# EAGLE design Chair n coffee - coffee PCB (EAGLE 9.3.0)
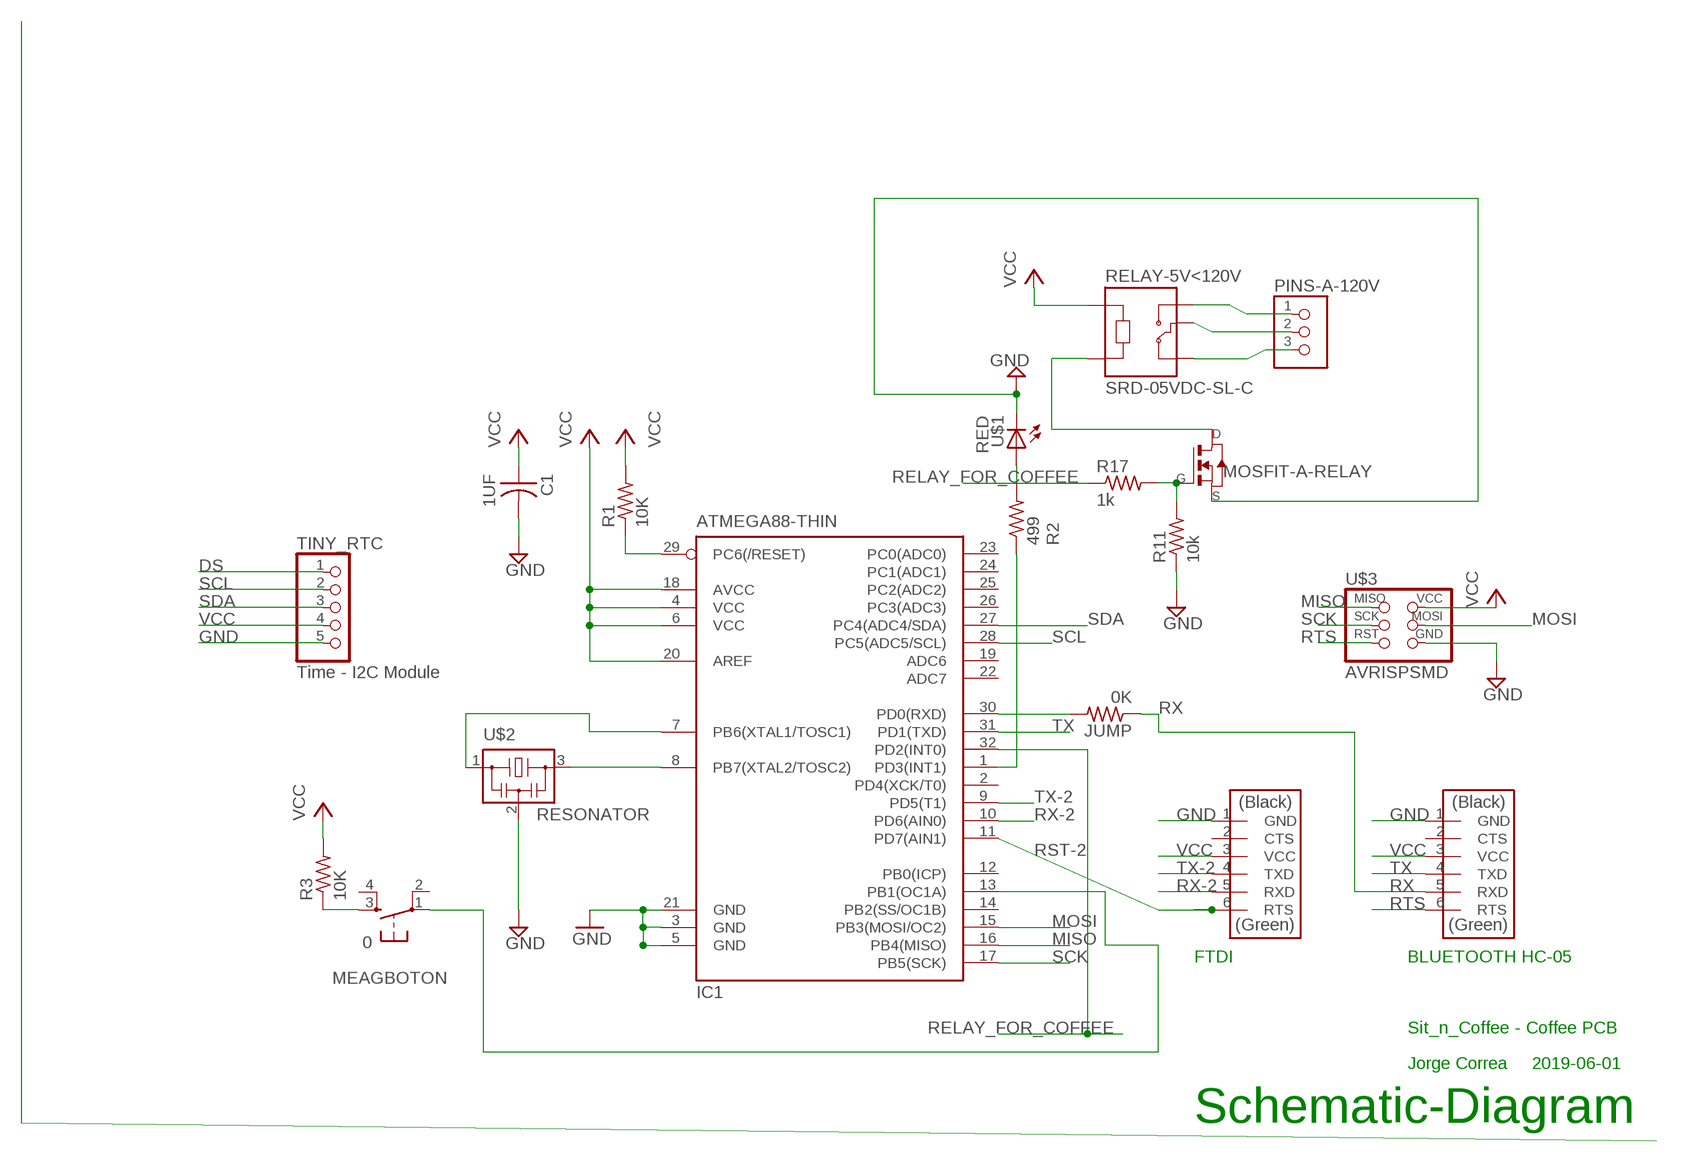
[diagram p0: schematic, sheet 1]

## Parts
C1  1UF  CAP-US1206FAB  [C1206FAB]
IC1  ATMEGA88-THIN  [TQFP32-08THIN]
JUMP  0K  RES-US1206FAB  [R1206FAB]
MEAGBOTON  0  6MM_SWITCH6MM_SWITCH  [6MM_SWITCH]
MOSFIT-A-RELAY  NMOSFETTO252  [TO252]
PINS-A-120V  TERM-1X03'-FABLAB'  [ED555DS-3DS]
R1  10K  RES-US1206FAB  [R1206FAB]
R2  499  RES-US1206FAB  [R1206FAB]
R3  10K  RES-US1206FAB  [R1206FAB]
R11  10k  RES-US1206FAB  [R1206FAB]
R17  1k  RES-US1206FAB  [R1206FAB]
RELAY-5V<120V  SRD-05VDC-SL-C  [RELAY_SRD-05VDC-SL-C]
TINY_RTC  Time - I2C Module  PINHD-1X5  [1X05]
U$1  RED  LEDFAB1206  [LED1206FAB]
U$2  RESONATOR  [EFOBM]
U$3  AVRISPSMD  [2X03SMD]
U$4  FTDI-SMD-HEADER  [1X06SMD]
U$5  FTDI-SMD-HEADER  [1X06SMD]

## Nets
DS: TINY_RTC.1
GND: C1.2 IC1.3(GND) IC1.5(GND) IC1.21(GND) MOSFIT-A-RELAY.2(S) R11.1 TINY_RTC.5 U$1.2(C) U$2.2 U$3.6(GND) U$4.1(GND) U$5.1(GND)
MISO: IC1.16(PB4(MISO)) U$3.1(MISO)
MOSI: IC1.15(PB3(MOSI/OC2)) U$3.4(MOSI)
N$1: IC1.8(PB7(XTAL2/TOSC2)) U$2.3
N$2: IC1.7(PB6(XTAL1/TOSC1)) U$2.1
N$3: IC1.29(PC6(/RESET)) R1.1
N$4: R2.2 U$1.1(A)
N$5: MEAGBOTON.3(S) R3.1
N$7: MOSFIT-A-RELAY.1(G) R11.2 R17.2
N$8: PINS-A-120V.2 RELAY-5V<120V.COM
N$9: PINS-A-120V.1 RELAY-5V<120V.NO
N$10: IC1.1(PD3(INT1)) R2.1
N$11: IC1.13(PB1(OC1A)) MEAGBOTON.1(P)
N$35: MOSFIT-A-RELAY.3(D) RELAY-5V<120V.A2
N$37: PINS-A-120V.3 RELAY-5V<120V.NC
RELAY_FOR_COFFEE: IC1.32(PD2(INT0)) R17.1
RST-2: IC1.11(PD7(AIN1)) U$4.6(RTS)
RTS: U$3.5(RST) U$5.6(RTS)
RX: IC1.30(PD0(RXD)) JUMP.1 JUMP.2 U$5.5(RXD)
RX-2: IC1.10(PD6(AIN0)) U$4.5(RXD)
SCK: IC1.17(PB5(SCK)) U$3.3(SCK)
SCL: IC1.28(PC5(ADC5/SCL)) TINY_RTC.2
SDA: IC1.27(PC4(ADC4/SDA)) TINY_RTC.3
TX: IC1.31(PD1(TXD)) U$5.4(TXD)
TX-2: IC1.9(PD5(T1)) U$4.4(TXD)
VCC: C1.1 IC1.4(VCC) IC1.6(VCC) IC1.18(AVCC) IC1.20(AREF) R1.2 R3.2 RELAY-5V<120V.A1 TINY_RTC.4 U$3.2(VCC) U$4.3(VCC) U$5.3(VCC)
Unconnected: IC1.2(PD4(XCK/T0)) IC1.12(PB0(ICP)) IC1.14(PB2(SS/OC1B)) IC1.19(ADC6) IC1.22(ADC7) IC1.23(PC0(ADC0)) IC1.24(PC1(ADC1)) IC1.25(PC2(ADC2)) IC1.26(PC3(ADC3)) MEAGBOTON.2(P1) MEAGBOTON.4(S1) U$4.2(CTS) U$5.2(CTS)

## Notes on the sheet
- FTDI | BLUETOOTH HC-05
- Sit_n_Coffee - Coffee PCB
- Jorge Correa | 2019-06-01
- Schematic-Diagram

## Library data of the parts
C1 = fab:CAP-US
IC1 = fab:ATMEGA88-THIN
JUMP R1-R3 R11 R17 = fab:RES-US: Resistor (US Symbol)
MEAGBOTON = fab:6MM_SWITCH: OMRON SWITCH
MOSFIT-A-RELAY = fab:NMOSFET: MOS FET
PINS-A-120V = fab:TERM-1X03: 3.5mm terminal block, 3 positions ED555-3DS as found in the fablab inventory. Made by Zaerc.
RELAY-5V<120V = SRD-05VDC-SL-C:SRD-05VDC-SL-C: 5V Trigger Relay Module For Arduino And Raspberry Pi 5V Trigger Relay Module For Arduino And Raspberry Pi; AVAILABILITY: Unavailable; DESCRIPTION: 5V Trigger Relay Module For Arduino And Raspberry Pi 5V Trigger Relay Module For Arduino And Raspberry Pi; MF: Songle Relay; MP: SRD-05VDC-SL-C; PACKAGE: None; PRICE: None
TINY_RTC = pinhead:PINHD-1X5: PIN HEADER
U$1 = fab:LED: LED
U$2 = fab:RESONATOR
U$3 = fab:AVRISP
U$4 U$5 = fab:FTDI-SMD-HEADER

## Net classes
0 default: width 0.508 mm, clearance 0.508 mm

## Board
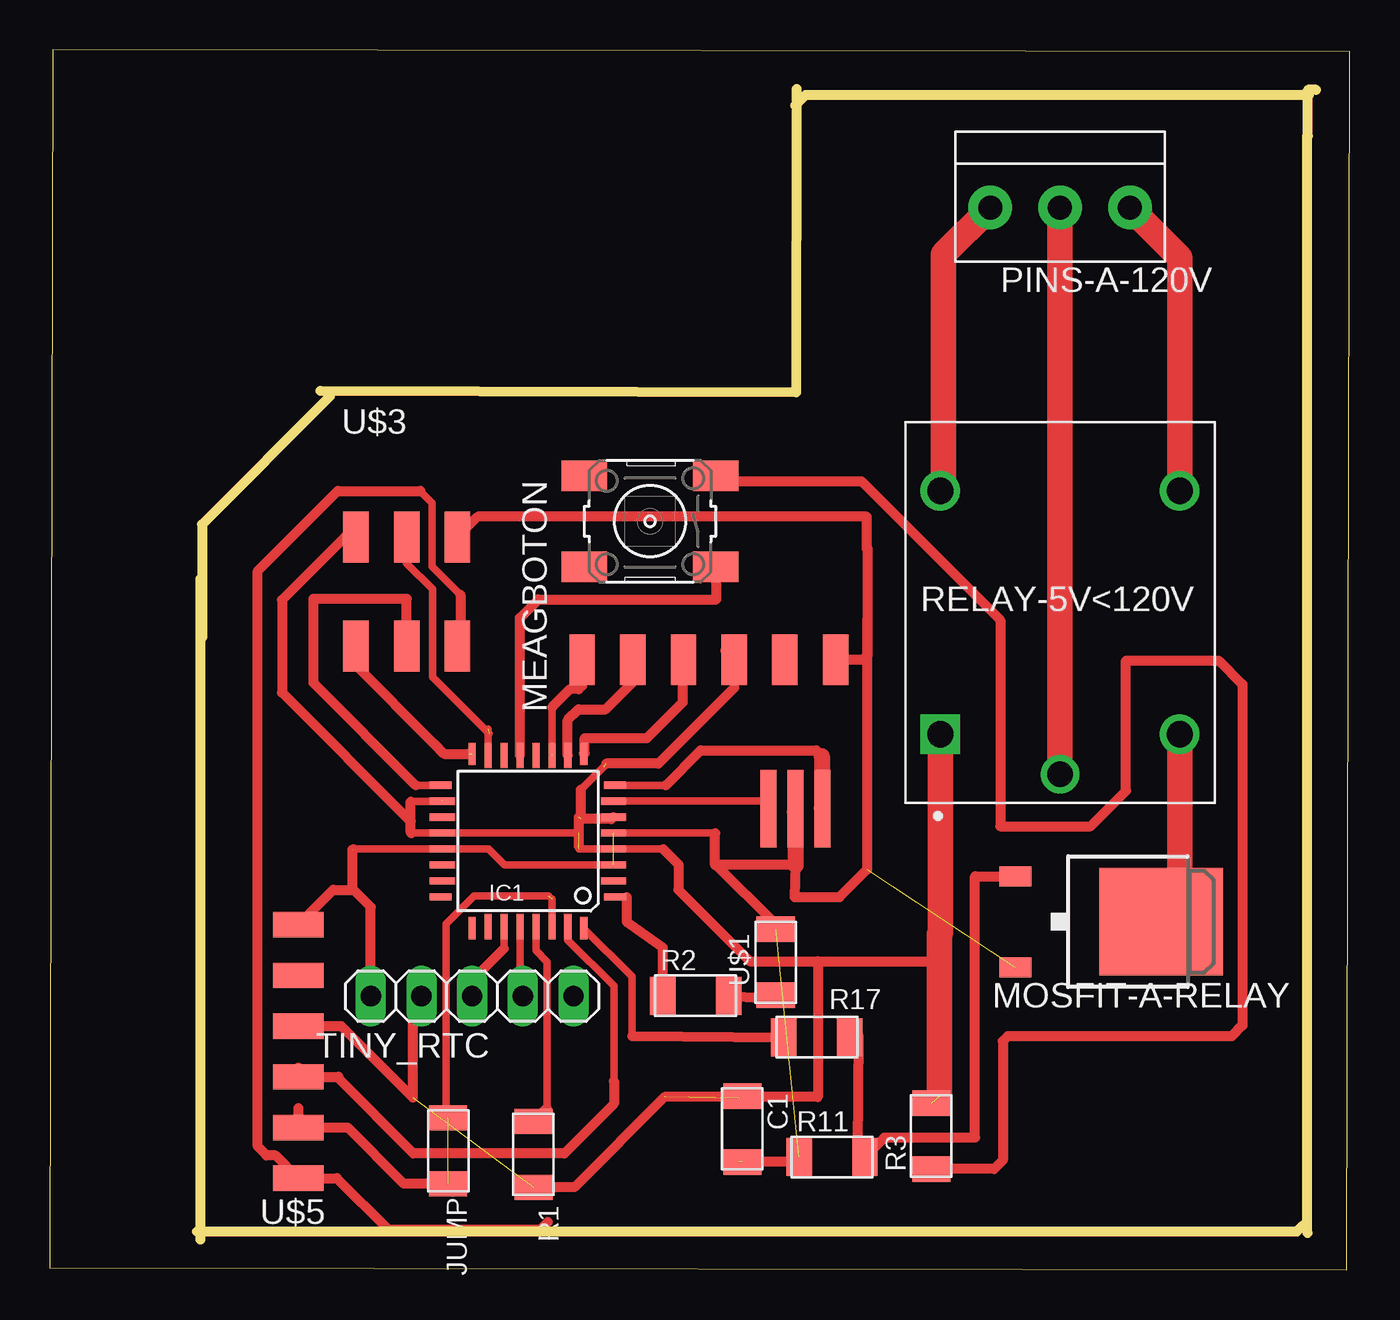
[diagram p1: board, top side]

Size 65.13 x 61.14 mm. Coordinates in mm from the lower left corner, seen from the top.
Outline: 0,0.1 64.98,0 65.13,61.04 0.15,61.14 0,0.1
Copper layers (1*16): Top 0.035mm / dielectric 1.5mm / Bottom 0.035mm
Design rules "default": minimum track width 6mil, minimum drill 0.35mm, track to track 6mil, track to pad 6mil, pad to pad 6mil, via to via 6mil, smd to smd 6mil, copper to edge 40mil, drill to drill 6mil, minimum pad ring 10mil, minimum via ring 8mil, stop-mask expansion 4mil, vias tented up to drill 0mil, thermal gap 10mil
Milling: 12 lines

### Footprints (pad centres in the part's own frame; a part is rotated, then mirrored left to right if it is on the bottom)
C1206FAB = smd 1.27 x 1.905: 1 -1.651,0; 2 1.651,0
TQFP32-08THIN = smd 1.118 x 0.356: 1 -4.369,2.8; 8 -4.369,-2.8; 17 4.369,-2.8; 24 4.369,2.8 | smd 1.27 x 0.356: 2 -4.293,2; 3 -4.293,1.2; 4 -4.293,0.4; 5 -4.293,-0.4; 6 -4.293,-1.2; 7 -4.293,-2; 18 4.293,-2; 19 4.293,-1.2; 20 4.293,-0.4; 21 4.293,0.4; 22 4.293,1.2; 23 4.293,2 | smd 0.356 x 1.118: 9 -2.8,-4.369; 16 2.8,-4.369; 25 2.8,4.369; 32 -2.8,4.369 | smd 0.356 x 1.27: 10 -2,-4.293; 14 1.2,-4.293; 15 2,-4.293; 26 2,4.293; 27 1.2,4.293; 31 -2,4.293 | smd 0.35 x 1.27: 11 -1.2,-4.293; 12 -0.4,-4.293; 13 0.4,-4.293; 28 0.4,4.293; 29 -0.4,4.293; 30 -1.2,4.293
R1206FAB = smd 1.27 x 1.905: 1 -1.651,0; 2 1.651,0
6MM_SWITCH = smd 2.286 x 1.524: 1 -3.302,2.286; 2 3.302,2.286; 3 -3.302,-2.286; 4 3.302,-2.286
TO252 = smd 1 x 1.6: 1 -2.28,-4.8; 2 2.28,-4.8 | smd 5.4 x 6.2: 3 0,2.5
ED555DS-3DS = drill 1.2 pad 2.184: 1 -3.5,0; 2 0,0; 3 3.5,0
RELAY_SRD-05VDC-SL-C = drill 1.32 square: A1 -6.1,6 | drill 1.32: A2 -6.1,-6; NC 6.1,6; NO 6.1,-6 | drill 1.29: COM -8.1,0
1X05 = drill 1.016 long: 1 -5.08,0; 2 -2.54,0; 3 0,0; 4 2.54,0; 5 5.08,0
LED1206FAB = smd 1.27 x 1.905: 1 -1.651,0; 2 1.651,0
EFOBM = smd 0.8 x 3.9: 1 -1.35,0; 2 0,0; 3 1.35,0
2X03SMD = smd 2.54 x 1.27: 1 -2.54,2.54; 2 2.92,2.54; 3 -2.54,0; 4 2.92,0; 5 -2.54,-2.54; 6 2.92,-2.54
1X06SMD = smd 2.54 x 1.27: 1 0,6.35; 2 0,3.81; 3 0,1.27; 4 0,-1.27; 5 0,-3.81; 6 0,-6.35

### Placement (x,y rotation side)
C1  34.7,7.06 270 top
IC1  23.95,21.49 180 top
JUMP  19.96,5.97 90 top
MEAGBOTON  30.07,37.52 180 top
MOSFIT-A-RELAY  53.19,17.45 270 top
PINS-A-120V  50.62,53.24 180 top
R1  24.23,5.79 270 top
R2  32.36,13.74 0 top
R3  44.17,6.71 90 top
R11  39.19,5.66 0 top
R17  38.43,11.66 0 top
RELAY-5V<120V  50.62,32.94 90 top
TINY_RTC  21.16,13.72 180 top
U$1  36.37,15.42 90 top
U$2  37.36,23.11 0 top
U$3  17.88,33.81 90 top
U$4  33.02,30.58 270 top
U$5  12.45,10.95 0 top

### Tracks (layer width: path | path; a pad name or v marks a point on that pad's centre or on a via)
GND  (5 unrouted)
  Top 0.381: IC1.5 33.34,21.89 | 15.22,21.09 IC1.21 21.99,21.09 22.79,20.29 IC1.3
  Top 0.508: R11.1 37.29,5.41 34.52,5.41 | 12.78,17.3 U$5.1 14.2,19.05 15.11,19.05 15.16,19.1 | 33.34,20.35 33.34,20.29 37.36,20.29 37.31,18.69 39.57,18.69 40.95,20.07 40.95,30.81 | 33.34,20.35 33.34,21.89 | 15.16,19.1 15.16,21.06 | 15.16,21.03 15.22,21.09 | 37.18,22.93 U$2.2 | U$3.6 21.44,37.74 40.92,37.74 40.92,36.14 40.97,36.14 40.97,30.81 | 40.95,32.61 40.95,30.81 | 40.95,30.81 40.97,30.81 | U$1.2 36.37,17.32 33.34,20.35 | TINY_RTC.5 16.08,18.19 15.16,19.1 | U$4.1 40.74,30.58 40.97,30.81
  Top 0.813: U$2.2 37.36,20.29
MISO  (1 unrouted)
  Top 0.508: U$3.1 15.34,30.28 19.18,26.44 19.24,26.37 19.76,25.86 21,25.86
MOSI  (1 unrouted)
  Top 0.381: 21.95,27.11 IC1.15 | 22,26.88 19.18,29.71 19.18,34.11 17.88,35.41 U$3.4
N$1
  Top 0.381: IC1.8 30.87,24.29
  Top 0.508: 30.87,24.29 32.61,26.04 38.41,26.04 38.69,25.75
  Top 0.813: 38.69,25.75 38.69,23.14 U$2.3
N$2
  Top 0.381: IC1.7 36.01,23.49
  Top 0.508: U$2.1 36.01,23.49
N$3
  Top 0.381: IC1.29 24.35,16 24.91,15.44 24.91,8.12
  Top 0.508: 24.91,8.12 R1.1
N$4
  Top 0.508: R2.2 35.69,13.64 36.25,13.64 U$1.1
N$5
  Top 0.508: MEAGBOTON.3 33.66,39.52 40.67,39.52 47.63,32.56 47.63,22.23 52.15,22.23 53.92,24 53.92,30.53 58.57,30.53 59.77,29.34 59.77,12.24 59.23,11.71 48.01,11.71 47.75,11.46 47.75,5.49 47.32,5.05 R3.1
N$7
  Top 0.508: R11.2 41.81,6.63 46.36,6.63 46.36,19.73 MOSFIT-A-RELAY.1 | 40.61,6.12 R11.2 | R11.2 40.47,6.04 40.53,11.73 R17.2
N$8
  Top 1.27: RELAY-5V<120V.COM PINS-A-120V.2
N$9
  Top 1.27: RELAY-5V<120V.NO 56.62,50.74 PINS-A-120V.1
N$10
  Top 0.381: IC1.1 28.91,18.69
  Top 0.508: 28.91,18.69 28.91,17.44 30.71,16.15 R2.1
N$11
  Top 0.508: MEAGBOTON.1 33.4,35.2 33.4,33.6 24.49,33.6 23.55,32.67 IC1.13
N$35
  Top 1.27: MOSFIT-A-RELAY.3 56.62,18.38 RELAY-5V<120V.A2
N$37
  Top 1.27: PINS-A-120V.3 44.78,50.9 44.78,39.2 RELAY-5V<120V.NC
RELAY_FOR_COFFEE
  Top 0.381: 29.18,11.72 29.17,14.71 IC1.32
  Top 0.508: 29.18,11.72 R17.1
RST-2  (1 unrouted)
  Top 0.381: 25.17,28.2 25.17,25.84
  Top 0.508: U$4.6 26.67,29.29 26.49,29.11 26.07,29.11 25.17,28.2
RTS
  Top 0.381: 20.57,33.82 19.15,35.24 19.15,38.44 18.55,39.04
  Top 0.508: 20.57,33.82 20.57,31.42 U$3.5 | 18.55,39.04 14.43,39.04 10.41,35.03 10.41,6.19 10.86,5.74 11.3,5.74 U$5.6 14.38,4.6 16.94,2.03 24.59,2.03 24.94,2.39
RX  (2 unrouted)
  Top 0.381: IC1.30 25.15,18.59 | 19.86,7.72 19.86,17.35 21.26,18.75 25,18.75
  Top 0.508: 12.45,8.1 U$5.5 14.91,7.14 17.73,4.32 JUMP.1 | JUMP.2 19.86,7.72
RX-2
  Top 0.508: IC1.10 25.95,27.55 26.49,28.09 27.84,28.09 29.21,29.46 U$4.5
SCK
  Top 0.381: IC1.17 18.33,24.29
  Top 0.508: U$3.3 17.88,33.63 13.21,33.63 13.21,29.41 18.33,24.29
SCL
  Top 0.381: IC1.28 23.55,13.86
  Top 0.508: 23.55,13.86 TINY_RTC.2
SDA
  Top 0.381: IC1.27 22.75,16.1
  Top 0.508: 22.75,16.1 21.16,14.51 TINY_RTC.3
TX
  Top 0.381: IC1.31 25.95,16.54 28.26,14.22 28.26,9.47
  Top 0.508: 12.45,10.13 U$5.4 14.45,9.68 14.41,9.64 18.21,5.84 25.78,5.84 28.26,8.32 28.26,9.47
TX-2
  Top 0.508: IC1.9 26.8,25.9 26.8,26.64 29.92,26.64 31.72,28.45 31.72,30.61 | 31.72,31.19 31.72,30.61 | 31.72,30.61 U$4.4
VCC  (8 unrouted)
  Top 0.381: 26.51,21.11 28.17,21.11 IC1.4 30.73,21.09 | 26.49,22.69 26.75,22.69 | 26.48,21.89 IC1.20 18.12,21.89 | 18.09,23.47 19.6,23.47 | 26.59,24.05 27.76,25.22
  Top 0.508: 44.58,16.84 44.58,16.61 | 44.27,27.1 RELAY-5V<120V.A1 | 38.48,15.47 44.58,15.47 | U$3.2 14.78,36.73 11.63,33.58 11.63,28.93 18.09,22.48 | 18.12,21.89 18.09,21.92 18.09,22.48 | 18.09,22.48 18.09,23.47 | 38.48,15.47 38.48,8.66 30.81,8.66 26.29,4.14 R1.2 | 30.73,21.09 31.5,20.32 31.5,19.05 35.08,15.47 38.48,15.47 | C1.1 34.57,8.59 34.57,8.51 | 26.49,22.69 26.49,21.25 26.51,21.24 | U$5.3 14.61,12.22 18.19,8.64 18.19,13.28 TINY_RTC.4 | 27.88,25.37 30.49,25.37 34.29,29.17 U$4.3 33.83,31.04 | 26.59,24.05 26.59,22.61 26.62,22.59 28.14,22.59 IC1.6
  Top 1.27: RELAY-5V<120V.A1 44.62,16.89 44.58,16.84 | 44.58,16.61 44.58,15.47 44.58,8.69 44.6,8.66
